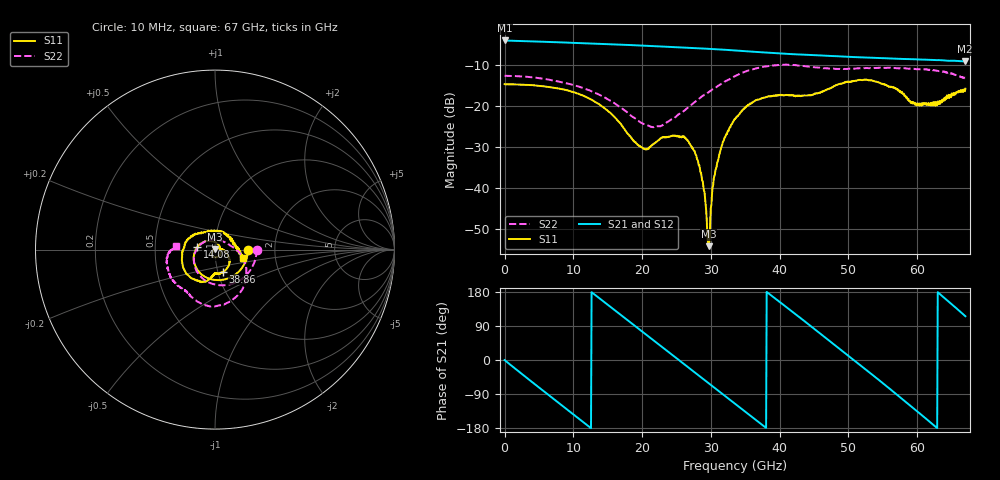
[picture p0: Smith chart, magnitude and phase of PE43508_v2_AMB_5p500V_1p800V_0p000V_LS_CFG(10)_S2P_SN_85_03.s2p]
!Keysight Technologies,N5227A,US51270237,A.10.43.00
!Date: Wednesday, August 22, 2018 17:07:33
!Correction: S11(Full 2 Port(1,3))
!S31(Full 2 Port(1,3))
!S13(Full 2 Port(1,3))
!S33(Full 2 Port(1,3))
!S2P File: Measurements: S11, S31, S13, S33:
# Hz S  dB  R 50
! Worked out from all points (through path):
!   801 points, 10 MHz to 67 GHz, reference 50 ohm
!   highest |S21| = -4.09 dB at 10 MHz (marker M1); lowest = -9.2 dB at 66.92 GHz (marker M2)
!   group delay of S21, straight-line fit = 39.6 ps
!   lowest |S11| = -54.1 dB at 29.65 GHz (marker M3), VSWR 1.00, Z = 49.9 + j0.171 ohm
!   |S11| at or under -10 dB: start of sweep to end of sweep
!   |S22| runs from -25.2 to -10.0 dB; largest |S21 - S12| = 0.003
!   S11 on the Smith chart (normalised r, x): 10 MHz: 1.45, -0.00; 14.08 GHz: 0.82, +0.02; 38.86 GHz: 1.06, -0.26; 67 GHz: 1.36, -0.13
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1e7  -14.71 -0.4  -4.09 -0.2  -4.09 -0.2  -12.67 -0.3
2.522125e9  -14.83 -35.8  -4.24 -36.9  -4.23 -36.9  -12.83 -28.5
5.70415e9  -15.24 -78.5  -4.40 -82.5  -4.40 -82.4  -13.40 -63.0
8.216275e9  -15.87 -111.4  -4.55 -118.2  -4.54 -118.2  -14.21 -89.7
1.123082e10  -17.38 -149.5  -4.73 -160.9  -4.72 -160.9  -15.53 -121.3
1.40779e10  -19.99 172.0  -4.91 158.8  -4.90 158.8  -17.53 -152.6
1.826478e10  -27.37 93.0  -5.20 99.7  -5.20 99.7  -22.20 151.1
2.044195e10  -30.54 19.6  -5.37 69.0  -5.37 69.0  -24.51 109.5
2.236791e10  -28.34 -41.3  -5.53 41.8  -5.52 41.9  -24.96 68.5
2.596862e10  -27.57 -105.9  -5.81 -8.9  -5.80 -8.8  -21.36 16.8
2.730842e10  -30.31 -123.5  -5.92 -27.8  -5.90 -27.7  -19.52 5.3
2.864822e10  -37.16 -148.4  -6.02 -46.8  -6.02 -46.7  -17.77 -4.4
2.965308e10  -54.10 120.0  -6.12 -61.0  -6.11 -60.9  -16.70 -11.3
3.099288e10  -33.49 16.0  -6.25 -80.0  -6.24 -79.9  -15.20 -21.1
3.3505e10  -23.25 -17.5  -6.51 -115.6  -6.50 -115.6  -12.76 -40.7
3.88642e10  -17.68 -69.5  -7.12 169.1  -7.13 169.1  -10.20 -81.1
4.472582e10  -17.33 -92.7  -7.63 86.6  -7.61 86.6  -10.56 -114.6
5.033624e10  -14.05 -118.4  -8.09 6.3  -8.09 6.3  -10.94 -129.3
5.586291e10  -15.37 175.1  -8.44 -74.0  -8.44 -74.3  -10.72 -147.4
6.180828e10  -19.49 53.5  -8.81 -163.1  -8.84 -163.3  -11.27 -168.3
6.691626e10  -16.44 -16.0  -9.17 116.9  -9.22 117.0  -13.14 175.6
6.7e10  -15.81 -17.0  -9.17 115.5  -9.21 115.7  -13.23 174.6
